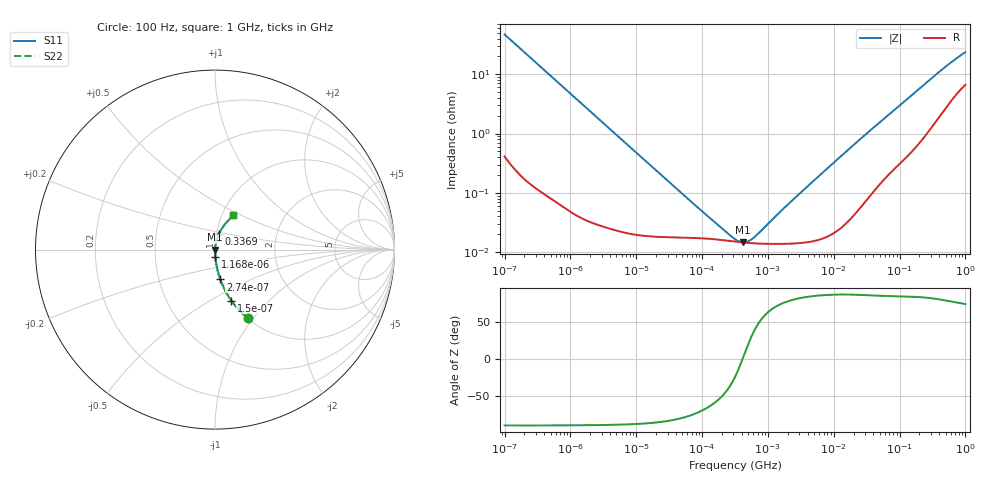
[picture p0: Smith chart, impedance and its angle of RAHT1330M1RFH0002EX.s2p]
! RAHT1330M1RFH0002EX  S-PARAMETER MODEL  (AEC-Q200 qualified)
! Model Generated by ELNA Corporation (http://www.ty-top.com)
! Version 1.0
! ELNA Control No. 201214
! Copyright (c) 2020 ELNA CO.,LTD. All Rights Reserved.
! Products Name : CONDUCTIVE POLYMER HYBRID ALUMINUM ELECTROLYTIC CAPACITORS
! Characteristics :
!  Capacitance  :  33uF  ,  Rated voltage  :  80V
!  Operating Temp. Range  :  -55 to +105 degC  ,  Endurance  :  10000hr at 105 degC
!  Dimension D  :  10mm  ,  Dimension L  :  10mm
! Frequency Range : 100Hz - 1GHz
! External Node Assignments :
!  1  o---| |---o  2
# MHz S RI R 50
!Freq[MHz].  S11 Real  S11 Imag  S21 Real  S21 Imag  S12 Real  S12 Imag  S22 Real  S22 Imag
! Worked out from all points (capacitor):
!   401 points, 100 Hz to 1 GHz, reference 50 ohm
!   read as one part in series: C = 33.9 uF near 108 Hz
!   lowest |Z| = 14.6 mohm at 419.3 kHz (marker M1)
!   series resonance near 413 kHz, so ESL is about 4.4 nH
!   S11 on the Smith chart (normalised r, x): 100 Hz: 1.01, -0.94; 150 Hz: 1.00, -0.63; 274 Hz: 1.00, -0.34; 1.168 kHz: 1.00, -0.08; 336.9 MHz: 1.03, +0.19; 1 GHz: 1.13, +0.45
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0.0001  0.1823 -0.3818  0.8177 0.3818  0.8177 0.3818  0.1823 -0.3818
0.00015  0.0912 -0.2842  0.9088 0.2842  0.9088 0.2842  0.0912 -0.2842
0.000274  0.0297 -0.1661  0.9703 0.1661  0.9703 0.1661  0.0297 -0.1661
0.000543  0.00819 -0.0859  0.9918 0.0859  0.9918 0.0859  0.00819 -0.0859
0.001168  0.00206 -0.0403  0.9979 0.0403  0.9979 0.0403  0.00206 -0.0403
0.001488  0.00138 -0.0317  0.9986 0.0317  0.9986 0.0317  0.00138 -0.0317
0.004241  0.000369 -0.0112  0.9996 0.0112  0.9996 0.0112  0.000369 -0.0112
0.022131  0.000186 -0.00215  0.9998 0.00215  0.9998 0.00215  0.000186 -0.00215
0.090678  0.000173 -0.00051  0.9998 0.00051  0.9998 0.00051  0.000173 -0.00051
0.316228  0.000151 -6.86e-05  0.9998 6.86e-05  0.9998 6.86e-05  0.000151 -6.86e-05
0.371535  0.000148 -2.72e-05  0.9999 2.72e-05  0.9999 2.72e-05  0.000148 -2.72e-05
0.419276  0.000146 3.92e-06  0.9999 -3.92e-06  0.9999 -3.92e-06  0.000146 3.92e-06
0.512861  0.000143 5.7e-05  0.9999 -5.7e-05  0.9999 -5.7e-05  0.000143 5.7e-05
0.627336  0.000141 0.000113  0.9999 -0.000113  0.9999 -0.000113  0.000141 0.000113
1.717908  0.000139 0.000524  0.9999 -0.000524  0.9999 -0.000524  0.000139 0.000524
4.704354  0.000154 0.00151  0.9998 -0.00151  0.9998 -0.00151  0.000154 0.00151
22.64644  0.000536 0.00723  0.9995 -0.00723  0.9995 -0.00723  0.000536 0.00723
69.9842  0.00252 0.021  0.9975 -0.021  0.9975 -0.021  0.00252 0.021
163.1173  0.00746 0.0462  0.9925 -0.0462  0.9925 -0.0462  0.00746 0.0462
336.8992  0.0226 0.0892  0.9774 -0.0892  0.9774 -0.0892  0.0226 0.0892
616.595  0.0567 0.1427  0.9433 -0.1427  0.9433 -0.1427  0.0567 0.1427
1000  0.1028 0.1907  0.8972 -0.1907  0.8972 -0.1907  0.1028 0.1907
